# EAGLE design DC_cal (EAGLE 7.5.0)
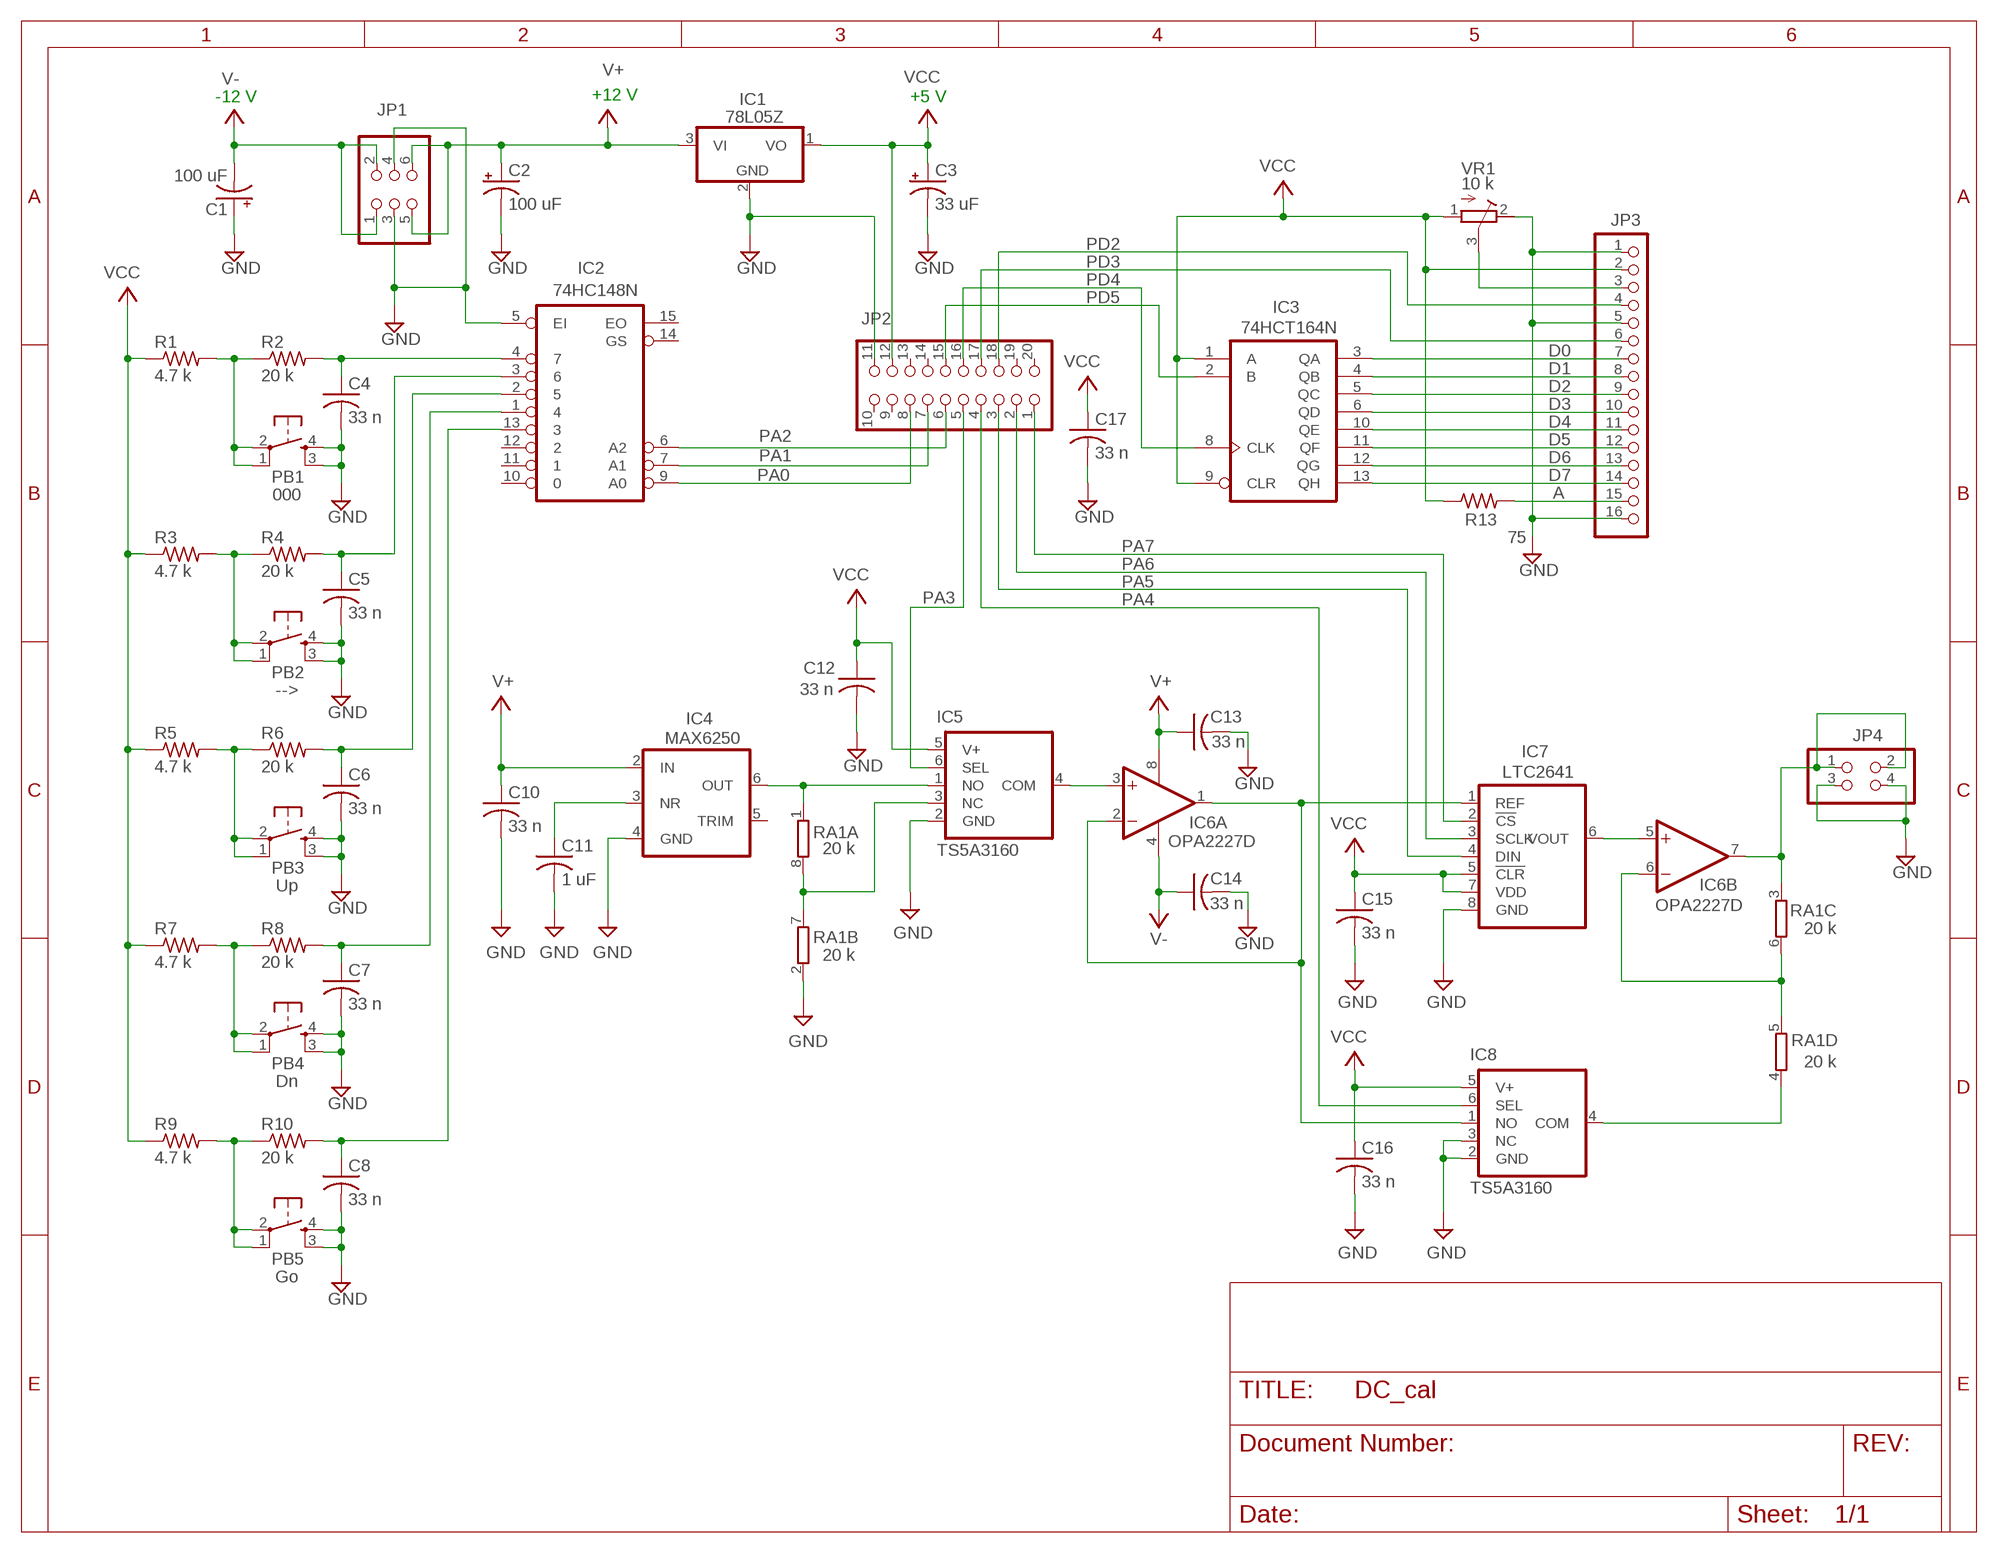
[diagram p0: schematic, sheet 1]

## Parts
C1  100 uF  CPOL-USE2.5-6  [E2,5-6]
C2  100 uF  CPOL-USE2.5-6  [E2,5-6]
C3  33 uF  CPOL-USE2.5-6  [E2,5-6]
C4  33 n  C-US025-024X044  [C025-024X044]
C5  33 n  C-US025-024X044  [C025-024X044]
C6  33 n  C-US025-024X044  [C025-024X044]
C7  33 n  C-US025-024X044  [C025-024X044]
C8  33 n  C-US025-024X044  [C025-024X044]
C10  33 n  C-US025-024X044  [C025-024X044]
C11  1 uF  C-US025-024X044  [C025-024X044]
C12  33 n  C-US025-024X044  [C025-024X044]
C13  33 n  C-US025-024X044  [C025-024X044]
C14  33 n  C-US025-024X044  [C025-024X044]
C15  33 n  C-US025-024X044  [C025-024X044]
C16  33 n  C-US025-024X044  [C025-024X044]
C17  33 n  C-US025-024X044  [C025-024X044]
IC1  78L05Z  [TO92]
IC2  74HC148N  [DIL16]
IC3  74HCT164N  [DIL14]
IC4  MAX6250  [SOIC8]
IC5  TS5A3160  [SOT-23]
IC6  OPA2227D  [SO08]
IC7  LTC2641  [MSOP8]
IC8  TS5A3160  [SOT-23]
JP1  PINHD-2X3  [2X03]
JP2  PIN_HDR_2X10  [MA10-2]
JP3  PINHD-1X16  [1X16]
JP4  PINHD-2X2  [2X02]
PB1  000  OMRON_B3F-1060  [B3F-10XX]
PB2  -->  OMRON_B3F-1060  [B3F-10XX]
PB3  Up  OMRON_B3F-1060  [B3F-10XX]
PB4  Dn  OMRON_B3F-1060  [B3F-10XX]
PB5  Go  OMRON_B3F-1060  [B3F-10XX]
R1  4.7 k  R-US_0204/5  [0204/5]
R2  20 k  R-US_0204/5  [0204/5]
R3  4.7 k  R-US_0204/5  [0204/5]
R4  20 k  R-US_0204/5  [0204/5]
R5  4.7 k  R-US_0204/5  [0204/5]
R6  20 k  R-US_0204/5  [0204/5]
R7  4.7 k  R-US_0204/5  [0204/5]
R8  20 k  R-US_0204/5  [0204/5]
R9  4.7 k  R-US_0204/5  [0204/5]
R10  20 k  R-US_0204/5  [0204/5]
R13  75  R-US_0207/10  [0207/10]
RA1  20 k  MORN  [MSOP8]
VR1  10 k  TRIM_RES  [TRIMMT93YB]

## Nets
A: JP3.15 R13.2
D0: IC3.3(QA) JP3.7
D1: IC3.4(QB) JP3.8
D2: IC3.5(QC) JP3.9
D3: IC3.6(QD) JP3.10
D4: IC3.10(QE) JP3.11
D5: IC3.11(QF) JP3.12
D6: IC3.12(QG) JP3.13
D7: IC3.13(QH) JP3.14
GND: C1.+ C2.- C3.- C4.2 C5.2 C6.2 C7.2 C8.2 C10.2 C11.2 C12.2 C13.2 C14.2 C15.2 C16.2 C17.2 IC1.2(GND) IC2.5(EI) IC4.4(GND) IC5.2(GND) IC7.8(GND) IC8.2(GND) IC8.3(NC) JP1.3 JP1.4 JP2.11 JP3.1 JP3.5 JP3.16 JP4.3 JP4.4 PB1.3 PB1.4 PB2.3 PB2.4 PB3.3 PB3.4 PB4.3 PB4.4 PB5.3 PB5.4 RA1.2 VR1.2
N$1: IC6.5(B:+IN) IC7.6(VOUT)
N$2: IC4.6(OUT) IC5.1(NO) RA1.1
N$3: IC5.3(NC) RA1.7 RA1.8
N$4: PB1.1 PB1.2 R1.2 R2.1
N$5: PB2.1 PB2.2 R3.2 R4.1
N$6: C4.1 IC2.4 R2.2
N$7: C5.1 IC2.3 R4.2
N$8: PB3.1 PB3.2 R5.2 R6.1
N$9: C6.1 IC2.2 R6.2
N$10: PB4.1 PB4.2 R7.2 R8.1
N$11: C7.1 IC2.1 R8.2
N$12: PB5.1 PB5.2 R9.2 R10.1
N$13: C8.1 IC2.13 R10.2
N$14: C11.1 IC4.3(NR)
N$17: IC6.7(B:OUT) JP4.1 JP4.2 RA1.3
N$21: IC6.6(B:-IN) RA1.5 RA1.6
N$35: IC5.4(COM) IC6.3(A:+IN)
N$36: IC6.1(A:OUT) IC6.2(A:-IN) IC7.1(REF) IC8.1(NO)
N$41: IC8.4(COM) RA1.4
PA0: IC2.9(A0) JP2.8
PA1: IC2.7(A1) JP2.7
PA2: IC2.6(A2) JP2.6
PA3: IC5.6(SEL) JP2.5
PA4: IC8.6(SEL) JP2.4
PA5: IC7.4(DIN) JP2.3
PA6: IC7.3(SCLK) JP2.2
PA7: IC7.2(!CS) JP2.1
PD2: JP2.18 JP3.4
PD3: JP2.17 JP3.6
PD4: IC3.8(CLK) JP2.16
PD5: IC3.2(B) JP2.15
V+: C2.+ C10.1 C13.1 IC1.3(VI) IC4.2(IN) IC6.8(P:V+) JP1.5 JP1.6
V-: C1.- C14.1 IC6.4(P:V-) JP1.1 JP1.2
VC: JP3.3 VR1.3
VCC: C3.+ C12.1 C15.1 C16.1 C17.1 IC1.1(VO) IC3.1(A) IC3.9(CLR) IC5.5(V+) IC7.5(!CLR) IC7.7(VDD) IC8.5(V+) JP2.12 JP3.2 R1.1 R3.1 R5.1 R7.1 R9.1 R13.1 VR1.1
Unconnected: IC2.10 IC2.11 IC2.12 IC2.14(GS) IC2.15(EO) IC4.5(TRIM) JP2.9 JP2.10 JP2.13 JP2.14 JP2.19 JP2.20

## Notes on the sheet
- -12 V | +12 V | +5 V

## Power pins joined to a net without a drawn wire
GND: IC2.8(GND) IC3.7(GND)
VCC: IC2.16(VCC) IC3.14(VCC)

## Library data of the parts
C1-C3 = rcl:CPOL-US: POLARIZED CAPACITOR, American symbol
C4-C8 C10-C17 = rcl:C-US: CAPACITOR, American symbol
IC1 = linear:78*: Positive VOLTAGE REGULATOR Source: http://cache.national.com/ds/LM/LM78L05.pdf http://www.fairchildsemi.com/ds/LM/LM7805.pdf
IC2 = 74xx-eu:74*148: 10-line to 4-line and 8-line to 3-line PRIORITY ENCODER
IC3 = 74xx-us:74*164: 8-bit parallel out SHIFT REGISTER
IC4 = zMyParts:MAX6250
IC5 IC8 = zMyParts:TS5A3160
IC6 = linear:OPA222*: High Precision, Low Noise OPERATIONAL AMPLIFIERS Source: http://focus.ti.com/lit/ds/symlink/opa227.pdf
IC7 = zMyParts:LTC2641
JP1 = pinhead:PINHD-2X3: PIN HEADER
JP2 = zMyParts:PIN_HDR_2X10
JP3 = pinhead:PINHD-1X16: PIN HEADER
JP4 = pinhead:PINHD-2X2: PIN HEADER
PB1-PB5 = zMyParts:OMRON_B3F-1060
R1-R10 R13 = rcl:R-US_: RESISTOR, American symbol
RA1 = zMyParts:MORN
VR1 = zMyParts:TRIM_RES

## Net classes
0 default: width 0.254 mm, drill 0.6 mm, clearance 0.203 mm

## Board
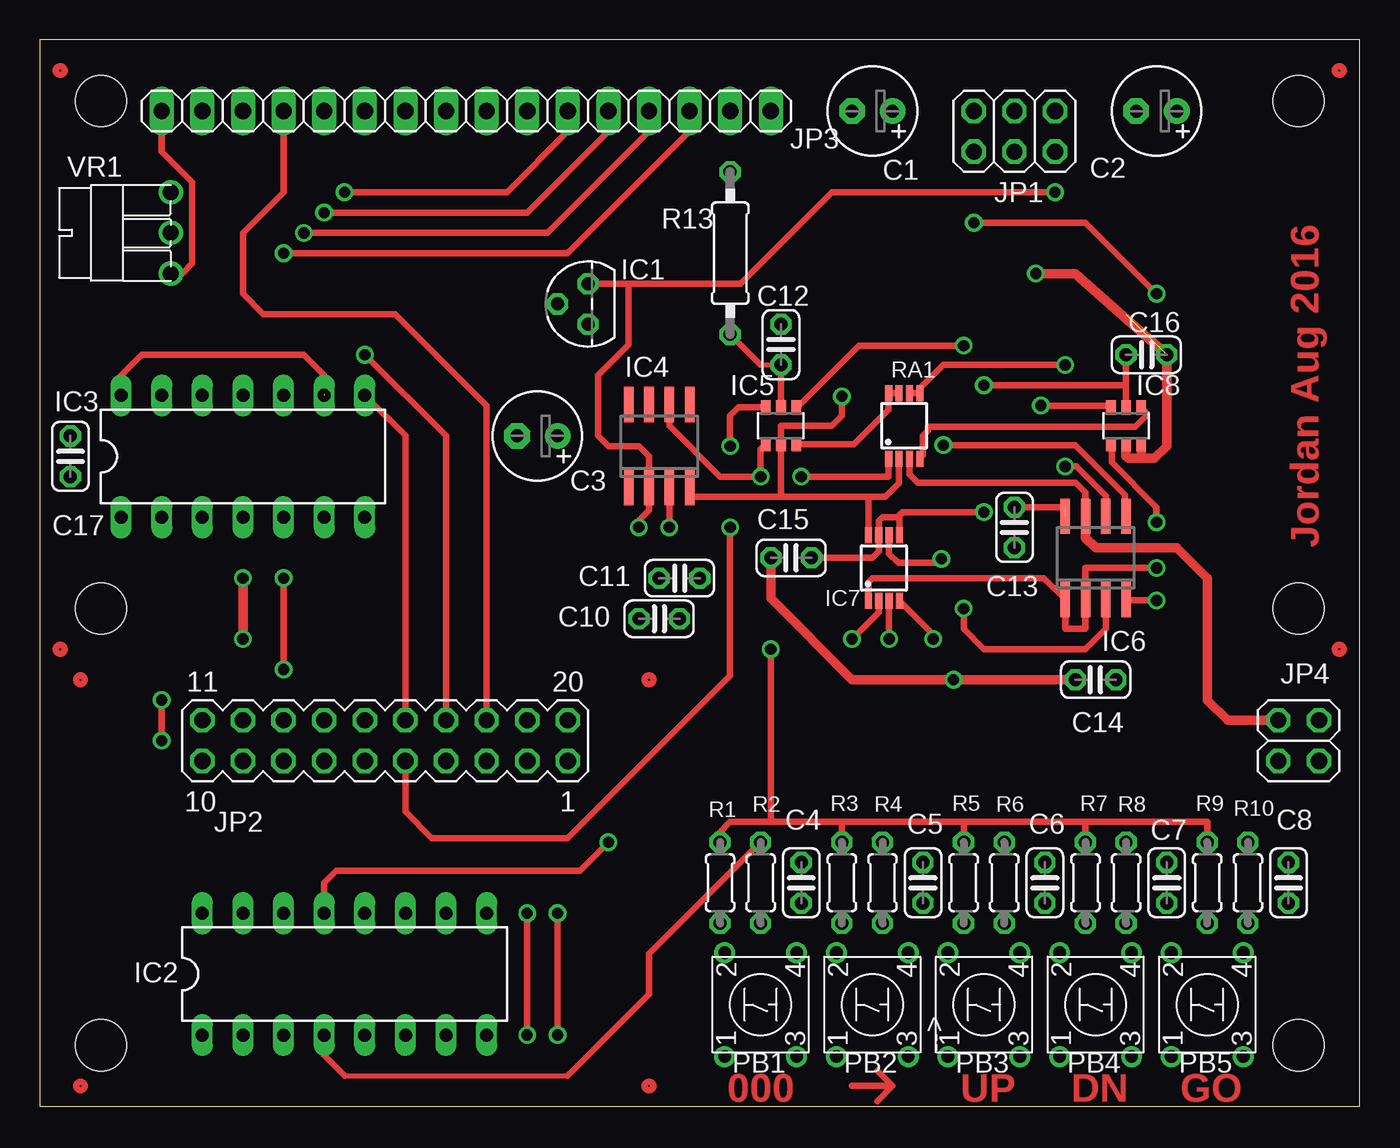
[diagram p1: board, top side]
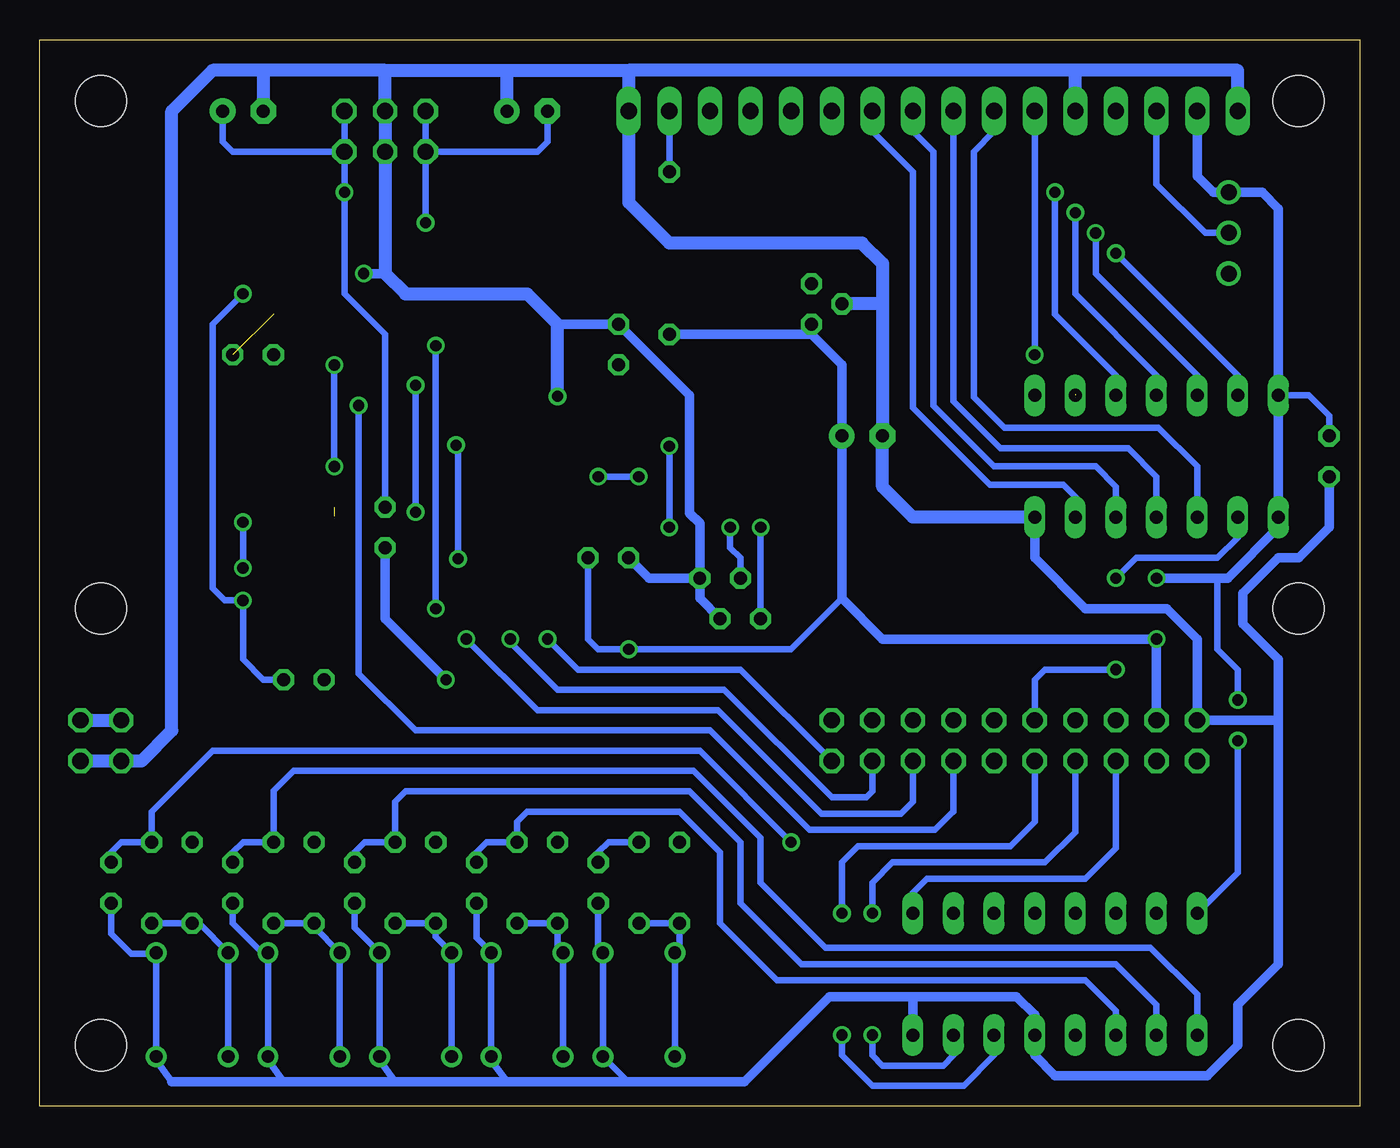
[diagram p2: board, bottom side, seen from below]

Size 82.55 x 66.67 mm. Coordinates in mm from the lower left corner, seen from the top.
Outline: 82.55,0 82.55,66.67 0,66.67 0,0 82.55,0
Copper layers (1*16): Top 0.035mm / dielectric 1.5mm / Bottom 0.035mm
Design rules "default *": minimum track width 10mil, minimum drill 24mil, track to track 8mil, track to pad 8mil, pad to pad 8mil, via to via 8mil, smd to smd 8mil, copper to edge 40mil, drill to drill 8mil, minimum pad ring 10mil, minimum via ring 8mil, stop-mask expansion 4mil, vias tented up to drill 0mil, thermal gap 10mil
Holes 3.2 mm at 3.81,62.87 3.81,31.11 78.74,3.81 3.81,3.81 78.74,62.87 78.74,31.11

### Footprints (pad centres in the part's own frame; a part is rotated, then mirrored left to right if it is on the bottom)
E2,5-6 = drill 0.813 pad 1.6: + -1.27,0 | drill 0.813 pad 1.6 octagon: - 1.27,0
C025-024X044 = drill 0.813 octagon: 1 -1.27,0; 2 1.27,0
TO92 = drill 0.813 octagon: 1 -1.27,0; 2 0,1.905; 3 1.27,0
DIL16 = drill 0.813 long: 1 -8.89,-3.81; 2 -6.35,-3.81; 3 -3.81,-3.81; 4 -1.27,-3.81; 5 1.27,-3.81; 6 3.81,-3.81; 7 6.35,-3.81; 8 8.89,-3.81; 9 8.89,3.81; 10 6.35,3.81; 11 3.81,3.81; 12 1.27,3.81; 13 -1.27,3.81; 14 -3.81,3.81; 15 -6.35,3.81; 16 -8.89,3.81
DIL14 = drill 0.813 long: 1 -7.62,-3.81; 2 -5.08,-3.81; 3 -2.54,-3.81; 4 0,-3.81; 5 2.54,-3.81; 6 5.08,-3.81; 7 7.62,-3.81; 8 7.62,3.81; 9 5.08,3.81; 10 2.54,3.81; 11 0,3.81; 12 -2.54,3.81; 13 -5.08,3.81; 14 -7.62,3.81
SOIC8 = smd 0.6 x 2.2: 1 -1.905,-2.6; 2 -0.635,-2.6; 3 0.635,-2.6; 4 1.905,-2.6; 5 1.905,2.6; 6 0.635,2.6; 7 -0.635,2.6; 8 -1.905,2.6
SOT-23 = smd 0.6 x 0.9: 1 -0.95,-1.15; 2 0,-1.15; 3 0.95,-1.15; 4 0.95,1.15; 5 0,1.15; 6 -0.95,1.15
SO08 = smd 0.6 x 2.2: 1 -1.905,-2.6; 2 -0.635,-2.6; 3 0.635,-2.6; 4 1.905,-2.6; 5 1.905,2.6; 6 0.635,2.6; 7 -0.635,2.6; 8 -1.905,2.6
MSOP8 = smd 0.45 x 1: 1 -0.885,-2.05; 2 -0.235,-2.05; 3 0.415,-2.05; 4 1.065,-2.05; 5 1.065,2.05; 6 0.415,2.05; 7 -0.235,2.05; 8 -0.885,2.05
2X03 = drill 1.016 octagon: 1 -2.54,-1.27; 2 -2.54,1.27; 3 0,-1.27; 4 0,1.27; 5 2.54,-1.27; 6 2.54,1.27
MA10-2 = drill 1.016 octagon: 1 11.43,-1.27; 2 8.89,-1.27; 3 6.35,-1.27; 4 3.81,-1.27; 5 1.27,-1.27; 6 -1.27,-1.27; 7 -3.81,-1.27; 8 -6.35,-1.27; 9 -8.89,-1.27; 10 -11.43,-1.27; 11 -11.43,1.27; 12 -8.89,1.27; 13 -6.35,1.27; 14 -3.81,1.27; 15 -1.27,1.27; 16 1.27,1.27; 17 3.81,1.27; 18 6.35,1.27; 19 8.89,1.27; 20 11.43,1.27
1X16 = drill 1.016 long: 1 -19.05,0; 2 -16.51,0; 3 -13.97,0; 4 -11.43,0; 5 -8.89,0; 6 -6.35,0; 7 -3.81,0; 8 -1.27,0; 9 1.27,0; 10 3.81,0; 11 6.35,0; 12 8.89,0; 13 11.43,0; 14 13.97,0; 15 16.51,0; 16 19.05,0
2X02 = drill 1.016 octagon: 1 -1.27,-1.27; 2 -1.27,1.27; 3 1.27,-1.27; 4 1.27,1.27
B3F-10XX = drill 0.8: 1 -3.25,2.25; 2 3.25,2.25; 3 -3.25,-2.25; 4 3.25,-2.25
0204/5 = drill 0.813 octagon: 1 -2.54,0; 2 2.54,0
0207/10 = drill 0.813 octagon: 1 -5.08,0; 2 5.08,0
TRIMMT93YB = drill 1: 1 4,2.54; 2 4,-2.54; 3 4,0

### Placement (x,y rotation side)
C1  52.07,62.23 180 top
C2  69.85,62.23 180 top
C3  31.11,41.91 180 top
C4  47.62,13.97 270 top
C5  55.24,13.97 270 top
C6  62.87,13.97 270 top
C7  70.48,13.97 270 top
C8  78.11,13.97 270 top
C10  38.73,30.48 0 top
C11  40.01,33.02 0 top
C12  46.35,47.62 90 top
C13  60.96,36.2 270 top
C14  66.04,26.67 180 top
C15  46.99,34.29 180 top
C16  69.22,46.99 0 top
C17  1.91,40.64 270 top
IC1  34.29,50.16 90 top
IC2  19.05,8.26 0 top
IC3  12.7,40.64 0 top
IC4  38.73,41.27 0 top
IC5  46.35,42.55 0 top
IC6  66.04,34.29 0 top
IC7  52.7,33.66 0 top
IC8  67.94,42.55 0 top
JP1  60.96,60.96 0 top
JP2  21.59,22.86 0 top
JP3  26.67,62.23 0 top
JP4  78.74,22.86 270 top
PB1  45.09,6.35 90 top
PB2  52.07,6.35 90 top
PB3  59.05,6.35 90 top
PB4  66.04,6.35 90 top
PB5  73.03,6.35 90 top
R1  42.55,13.97 270 top
R2  45.09,13.97 90 top
R3  50.16,13.97 270 top
R4  52.7,13.97 90 top
R5  57.78,13.97 270 top
R6  60.33,13.97 90 top
R7  65.41,13.97 270 top
R8  67.94,13.97 90 top
R9  73.03,13.97 270 top
R10  75.56,13.97 90 top
R13  43.18,53.34 90 top
RA1  53.98,42.55 0 top
VR1  4.19,54.61 0 top

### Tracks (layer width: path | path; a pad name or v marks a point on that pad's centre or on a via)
A
  Bottom 0.406: JP3.15 R13.2
D0
  Bottom 0.406: JP3.7 22.86,60.96 24.13,59.69 24.13,44.32 22.23,42.42 12.57,42.42 10.16,40.01 IC3.3
D1
  Bottom 0.406: JP3.8 25.4,44.07 22.48,41.15 14.48,41.15 12.7,39.37 IC3.4
D2
  Bottom 0.406: IC3.5 15.24,38.73 16.51,40.01 22.86,40.01 26.67,43.81 26.67,59.69 27.94,60.96 JP3.9
D3
  Bottom 0.406: IC3.6 17.78,38.1 18.54,38.86 23.11,38.86 27.94,43.69 27.94,58.42 30.48,60.96 JP3.10
D4  (via drill 0.7)
  Top 0.406: v19.05,57.15 29.21,57.15 33.02,60.96 JP3.11
  Bottom 0.406: v19.05,57.15 19.05,49.53 15.24,45.72 IC3.10
D5  (via drill 0.7)
  Top 0.406: JP3.12 35.56,60.96 30.48,55.88 v17.78,55.88
  Bottom 0.406: v17.78,55.88 17.78,50.8 12.7,45.72 IC3.11
D6  (via drill 0.7)
  Top 0.406: JP3.13 38.1,60.96 31.75,54.61 v16.51,54.61
  Bottom 0.406: IC3.12 10.16,45.72 16.51,52.07 v16.51,54.61
D7  (via drill 0.7)
  Top 0.406: JP3.14 40.64,60.96 33.02,53.34 v15.24,53.34
  Bottom 0.406: v15.24,53.34 7.62,45.72 IC3.13
GND  (via drill 0.7)  (1 unrouted)
  Top 0.305: IC8.3
  Top 0.406: VR1.2 8.89,52.07 9.53,52.7 9.53,57.78 7.62,59.69 JP3.1 | IC4.4 40.64,38.1 46.35,38.1 | 46.35,38.1 IC5.2 46.35,42.55 49.53,42.55 50.16,43.18 v50.16,44.39 | 46.35,38.1 51.82,38.1 | 51.82,38.1 IC7.8 | 51.82,38.1 52.9,38.1 53.74,38.94 RA1.2 | 68.07,40.51 67.94,40.64
  Top 0.61: 68.9,40.51 69.72,40.51 70.48,41.27 C16.2 64.77,52.07 v62.29,52.07 | 68.9,40.51 IC8.3 | 68.9,40.51 68.07,40.51 | 67.94,40.64 IC8.2 | C15.2 45.72,31.75 50.8,26.67 v57.15,26.67 C14.2
  Bottom 0.305: 47.32,9.58 PB1.4
  Bottom 0.406: PB3.3 PB3.4 | PB4.3 PB4.4 | PB5.3 PB5.4 | 47.32,9.58 47.32,3.12 PB1.3 45.76,1.52 45.72,1.52 | C4.2 47.62,9.89 PB1.4 | PB2.4 PB2.3 | C8.2 78.11,10.79 76.83,9.53 75.35,9.53 PB5.4 | C7.2 70.48,11.43 68.58,9.53 68.36,9.53 PB4.4 | C6.2 62.87,11.16 PB3.4 | C5.2 55.24,10.53 PB2.4 | PB2.4 54.32,2.88 53.34,1.52 | PB3.4 61.3,2.88 60.33,1.52 | PB4.4 68.29,2.88 67.31,1.52 | PB5.4 75.28,2.88 74.3,1.52
  Bottom 0.61: 27.94,6.86 IC2.8 | 5.08,24.13 JP2.11 10.16,29.21 12.06,31.11 17.14,31.11 20.32,34.29 IC3.7 | C17.2 1.91,36.2 3.81,34.29 5.08,34.29 7.3,32.07 7.3,30.16 5.08,27.94 5.08,24.13 | 50.16,48.9 C12.2 41.91,44.45 41.91,37.08 41.27,36.45 C11.2 | 5.08,24.13 5.08,8.89 7.62,6.35 7.62,3.81 9.53,1.91 19.05,1.91 20.32,3.17 IC2.5 20.32,5.71 21.46,6.86 27.94,6.86 | C11.2 41.27,31.75 C10.2 | v62.29,52.07 60.96,52.07 | C13.2 60.96,30.48 v57.15,26.67 | 27.94,6.86 33.15,6.86 38.48,1.52 45.72,1.52 | C11.2 44.45,33.02 C15.2 | 45.76,1.52 53.34,1.52 60.33,1.52 67.31,1.52 74.3,1.52
  Bottom 0.813: JP3.1 7.62,64.77 17.78,64.77 | JP3.5 17.78,64.77 | 17.78,64.77 45.72,64.77 | 45.72,64.77 JP3.16 45.72,56.52 43.18,53.98 31.11,53.98 29.84,52.7 29.84,50.16 | JP4.4 JP4.3 76.2,21.59 74.3,23.5 74.3,62.23 71.75,64.77 68.58,64.77 | 60.96,64.77 53.34,64.77 | 53.34,64.77 45.72,64.77 | IC3.7 27.94,36.83 29.84,38.73 C3.- 29.84,50.16 | C1.+ 53.34,64.77 | 60.96,64.77 JP1.4 JP1.3 60.96,52.07 59.69,50.8 52.07,50.8 50.16,48.9 v50.16,44.39 | 60.96,64.77 68.58,64.77 | 68.58,64.77 C2.- | 29.84,50.16 IC1.2
N$1  (via drill 0.7)
  Top 0.305: IC6.5 67.88,36.95
  Top 0.406: v56.52,41.34 64.77,41.34 67.88,38.23 67.88,36.95 | v56.39,34.23 56.13,33.97 53.69,33.97 53.12,34.54 IC7.6
  Bottom 0.305: v56.52,41.34 56.39,41.21
  Bottom 0.406: 56.39,41.21 v56.39,34.23
N$2  (via drill 0.7)
  Top 0.406: IC4.6 39.37,42.55 42.55,39.37 v45.09,39.37 45.09,41.08 IC5.1 | RA1.1 53.09,39.37 v47.62,39.37
  Bottom 0.406: v47.62,39.37 v45.09,39.37
N$3
  Top 0.406: RA1.7 RA1.8 53.09,43.56 50.92,41.4 IC5.3
N$4
  Bottom 0.406: R2.1 R1.2 42.55,9.89 PB1.2 PB1.1
N$5
  Bottom 0.406: R4.1 R3.2 50.16,9.95 PB2.2 PB2.1
N$6
  Top 0.305: 19.05,1.91 33.02,1.91
  Top 0.406: IC2.4 17.78,3.17 19.05,1.91 | 33.02,1.91 38.1,6.99 38.1,9.53 R2.2
  Bottom 0.406: C4.1 47.62,15.88 46.99,16.51 R2.2
N$7
  Bottom 0.406: C5.1 55.24,15.88 54.61,16.51 R4.2 52.7,17.78 52.07,18.41 42.55,18.41 40.01,15.88 40.01,11.43 36.45,7.87 17.14,7.87 15.24,5.97 IC2.3
N$8
  Bottom 0.406: R6.1 R5.2 57.78,10.58 PB3.2 | PB3.1 PB3.2 | 56.88,9.53 PB3.2
N$9
  Bottom 0.406: C6.1 62.87,15.88 62.23,16.51 R6.2 60.33,19.05 59.69,19.68 41.91,19.68 38.73,16.51 38.73,12.7 34.92,8.89 15.24,8.89 12.7,6.35 IC2.2
N$10
  Bottom 0.406: R8.1 R7.2 65.41,11.21 PB4.2 PB4.1
N$11
  Bottom 0.406: C7.1 70.48,15.88 69.85,16.51 R8.2 67.94,19.71 66.67,20.98 41.66,20.98 37.47,16.79 37.47,13.97 33.4,9.91 13.08,9.91 10.16,6.99 IC2.1
N$12
  Bottom 0.406: R10.1 R9.2 72.61,11.43 PB5.2 PB5.1
N$13  (via drill 0.7)
  Top 0.406: v35.56,16.51 33.78,14.73 18.54,14.73 17.78,13.97 IC2.13
  Bottom 0.406: C8.1 78.11,15.88 77.47,16.51 R10.2 75.56,18.41 71.75,22.23 41.27,22.23 v35.56,16.51
N$14  (via drill 0.7)
  Top 0.406: v39.37,36.2 IC4.3
  Bottom 0.406: v39.37,36.2 39.37,34.92 38.73,34.29 C11.1
N$17
  Top 0.406: IC6.7 65.41,38.39 64.8,38.99 54.93,38.99 54.39,39.53 RA1.3
  Top 0.61: JP4.1 74.3,24.13 73.03,25.4 73.03,33.02 71.12,34.92 66.04,34.92 65.41,35.56 IC6.7
  Bottom 0.813: JP4.2 JP4.1
N$18
  Top 0.406: 50.8,1.27 53.34,1.27 | 52.39,2.22 53.34,1.27 | 53.34,1.27 52.39,0.32
N$21  (via drill 0.7)
  Top 0.305: RA1.5 55.04,44.88
  Top 0.406: IC6.6 66.67,38.16 64.83,40.01 v64.14,40.01 | RA1.6 RA1.5 | v64.14,46.35 56.52,46.35 55.04,44.88
  Bottom 0.406: v64.14,46.35 v64.14,40.01
N$35  (via drill 0.7)
  Top 0.305: IC5.4 47.51,43.7 47.51,43.82
  Top 0.406: v57.78,47.56 51.24,47.56 47.51,43.82 | v57.78,31.11 57.78,29.84 59.05,28.57 65.41,28.57 66.67,29.84 IC6.3
  Bottom 0.406: v57.78,47.56 v57.78,31.11
N$36  (via drill 0.7)
  Top 0.305: 67.06,40.33 67.06,40.32 67.06,40.26 | 67.06,41.33 IC8.1
  Top 0.406: v69.85,36.51 69.85,37.47 67.06,40.26 | v69.85,33.66 65.41,33.66 IC6.2 65.41,29.84 64.14,29.84 IC6.1 62.8,33.02 52.07,33.02 51.82,32.77 IC7.1 | 67.06,40.33 67.06,41.33
  Bottom 0.406: v69.85,36.51 v69.85,33.66
N$41
  Top 0.305: 55.24,40.7 RA1.4
  Top 0.406: IC8.4 69.22,43.38 69.22,43.18 68.52,42.48 55.56,42.48 55.56,42.23 55.24,41.91 55.24,40.7
PA0
  Bottom 0.406: IC2.9 27.94,13.34 27.05,14.22 17.14,14.22 15.24,16.13 JP2.8
PA1  (via drill 0.7)
  Top 0.406: v30.48,4.45 v30.48,12.06
  Bottom 0.406: IC2.7 25.4,3.17 26.04,2.54 29.84,2.54 30.48,3.17 v30.48,4.45 | v30.48,12.06 30.48,13.97 29.21,15.24 19.68,15.24 17.78,17.14 JP2.7
PA2  (via drill 0.7)
  Top 0.406: v32.38,4.45 v32.38,12.06
  Bottom 0.406: IC2.6 22.86,3.17 24.77,1.27 30.48,1.27 32.38,3.17 v32.38,4.45 | v32.38,12.06 32.38,15.24 31.37,16.26 21.84,16.26 20.32,17.78 JP2.6
PA3  (via drill 0.7)
  Top 0.406: v43.18,36.2 43.18,26.92 33.02,16.76 24.51,16.76 22.86,18.41 JP2.5 | IC5.6 43.7,43.7 43.18,43.18 v43.18,41.27
  Bottom 0.406: v43.18,41.27 v43.18,36.2
PA4  (via drill 0.7)
  Top 0.305: 66.88,43.81 IC8.6
  Top 0.406: v62.61,43.81 66.88,43.81
  Bottom 0.406: v62.61,43.81 62.61,27.05 59.05,23.5 40.64,23.5 34.42,17.27 26.57,17.27 25.43,18.41 25.4,18.41 JP2.4
PA5  (via drill 0.7)
  Top 0.406: v55.88,29.21 55.88,29.5 IC7.4
  Bottom 0.406: v55.88,29.21 51.44,24.77 40.13,24.77 33.66,18.29 28.7,18.29 27.94,19.05 JP2.3
PA6  (via drill 0.7)  (1 unrouted)
  Top 0.406: v53.12,29.21 53.12,29.65 | IC7.3 53.12,29.66
  Bottom 0.406: v53.12,29.21 53.12,28.99 50.16,26.04 39.75,26.04 33.02,19.3 30.86,19.3 30.48,19.68 JP2.2
PA7  (via drill 0.7)
  Top 0.406: IC7.2 52.47,30.88 v50.8,29.21
  Bottom 0.406: JP2.1 38.73,27.3 48.9,27.3 v50.8,29.21
PD2
  Top 0.406: JP2.18 27.94,43.81 22.23,49.53 13.97,49.53 12.7,50.8 12.7,54.61 15.24,57.15 JP3.4
PD3  (via drill 0.7)
  Top 0.406: JP2.17 25.4,41.91 v20.32,46.99
  Bottom 0.406: JP3.6 v20.32,46.99
PD4
  Top 0.406: JP2.16 22.86,41.91 IC3.8
PD5  (via drill 0.7)
  Top 0.406: v15.24,33.02 v15.24,27.3
  Bottom 0.406: JP2.15 20.32,26.67 19.68,27.3 v15.24,27.3 | v15.24,33.02 13.97,34.29 8.89,34.29 7.62,35.56 IC3.2
V+  (via drill 0.7)  (1 unrouted)
  Top 0.406: IC1.3 36.83,51.44 | 36.83,51.44 43.81,51.44 49.53,57.15 v63.5,57.15 | C13.1 64.14,37.47 | 36.83,51.44 36.83,47.62 34.92,45.72 34.92,41.91 35.56,41.27 37.47,41.27 38.1,40.64 IC4.2 38.1,37.27 37.47,36.64 v37.47,36.2
  Bottom 0.406: JP1.6 JP1.5 | C2.+ 71.12,60.33 70.48,59.69 JP1.5 | C10.1 v37.47,36.2 | JP1.5 v63.5,57.15 63.5,50.8 60.96,48.26 C13.1
V-  (via drill 0.7)
  Top 0.305: v69.85,31.62
  Top 0.406: v69.85,31.62 68.01,31.62 IC6.4 | v58.42,55.24 65.41,55.24 v69.85,50.8
  Bottom 0.305: 69.91,31.62 v69.85,31.62
  Bottom 0.406: JP1.2 JP1.1 | C1.- 50.8,60.33 51.44,59.69 JP1.1 | v69.85,50.8 71.75,48.9 71.75,32.38 70.99,31.62 69.91,31.62 | JP1.1 v58.42,55.24 | v69.85,31.62 69.85,27.94 68.58,26.67 C14.1
VC
  Bottom 0.406: JP3.3 12.7,57.66 9.65,54.61 VR1.3
VCC  (via drill 0.7)  (1 unrouted)
  Top 0.305: 45.09,46.35 C12.1 | 53.77,36.94 53.77,36.83
  Top 0.406: R5.1 57.78,17.78 | 57.78,17.78 50.16,17.78 | 50.16,17.78 R3.1 | R7.1 65.41,17.78 | 65.41,17.78 57.78,17.78 | R9.1 73.03,17.78 65.41,17.78 | 45.72,17.78 50.16,17.78 | 17.78,44.53 17.78,45.72 16.51,46.99 6.35,46.99 5.08,45.72 IC3.14 | R1.1 42.55,17.14 43.18,17.78 45.72,17.78 | 45.72,17.78 v45.72,28.57 | v7.62,22.86 v7.62,25.4 | IC5.5 C12.1 | v59.05,37.15 53.98,37.15 53.77,36.94 | R13.1 45.09,46.35 | IC7.5 53.77,36.83 52.7,36.83 52.47,36.59 IC7.7 52.47,34.69 52.07,34.29 C15.1 | v59.05,45.09 67.94,45.09 | 67.94,45.09 IC8.5 | 67.94,45.09 C16.1
  Top 0.61: v12.7,33.02 v12.7,29.21
  Bottom 0.406: v7.62,25.4 7.62,27.3 8.89,28.57 8.89,33.02 | C17.1 1.91,43.18 3.17,44.45 IC3.14 | v59.05,37.15 v59.05,45.09 | C15.1 48.26,29.21 47.62,28.57 v45.72,28.57 35.56,28.57 32.38,31.75 | v7.62,22.86 7.62,14.61 IC2.16
  Bottom 0.61: 34.29,48.26 R13.1 | JP3.2 10.16,58.17 9.14,57.15 VR1.1 6.1,57.15 5.08,56.13 IC3.14 IC3.1 5.08,36.2 8.26,33.02 8.89,33.02 v12.7,33.02 | JP2.12 v12.7,29.21 29.84,29.21 32.38,31.75 C3.+ 32.38,46.35 34.29,48.26 | 34.29,48.26 IC1.1
(copper drawn outside any net)
  shapes: Top circle x8

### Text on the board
Top: Jordan Aug 2016 | 000 | UP | DN | GO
